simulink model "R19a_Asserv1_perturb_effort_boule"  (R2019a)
settings: Solver=ode15s  StartTime=0.0  StopTime=1  RelTol=1e-3  EnableMultiTasking=on
undefined symbols (not defined in the file): deg, kg, m, manette1_Défaut_sldprt, manette2_Défaut_sldprt, mm, N, rad, s, sigbuilder_block, STL, X, Y, Z
libraries: sm_lib x460, fl_lib x45, nesl_utility x23, simulink x3
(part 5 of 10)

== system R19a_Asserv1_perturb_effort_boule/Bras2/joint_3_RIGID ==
  AXE_BRAS_1_RIGID : Subsystem
  ReferenceFrame : sm_lib/Frames and Transforms/Reference Frame
  Transform : sm_lib/Frames and Transforms/Rigid Transform  TranslationMethod=Cartesian  TranslationStandardOffset=0  TranslationLengthUnit=mm  TranslationStandardAxis=+Z  TranslationCartesianOffset=[-182.62772197331239 126.3991346976174 -143.1183707091507]  TranslationROffset=0  TranslationROffsetUnits=m  TranslationZOffset=0  TranslationZOffsetUnits=m  TranslationThetaOffset=0  TranslationThetaOffsetUnits=deg  RotationMethod=ArbitraryAxis  RotationAngleUnits=rad  RotationStandardAxis=+Z  RotationAngle=2.0943951023931953  RotationArbitraryAxis=[0.57735026918962584 0.57735026918962584 0.57735026918962584]  FollAlignAxisA=+X  BaseAlignAxisA=+Y  FollAlignAxisB=+Y  BaseAlignAxisB=+Z  RotationSequenceAxes=FollowerAxes  RotationSequence=XYX  RotationSequenceAngles=[0 0 0]  RotationSequenceAnglesUnits=deg  RotationMatrix=[1 0 0; 0 1 0; 0 0 1]
  Transform1 : sm_lib/Frames and Transforms/Rigid Transform  TranslationMethod=Cartesian  TranslationStandardOffset=0  TranslationLengthUnit=mm  TranslationStandardAxis=+Z  TranslationCartesianOffset=[-181.62772197331239 116.1902983931664 -133.8263224253264]  TranslationROffset=0  TranslationROffsetUnits=m  TranslationZOffset=0  TranslationZOffsetUnits=m  TranslationThetaOffset=0  TranslationThetaOffsetUnits=deg  RotationMethod=ArbitraryAxis  RotationAngleUnits=rad  RotationStandardAxis=+Z  RotationAngle=1.9754511492118267  RotationArbitraryAxis=[-0.53149434051907762 -0.5314943405190774 -0.65956616953296032]  FollAlignAxisA=+X  BaseAlignAxisA=+Y  FollAlignAxisB=+Y  BaseAlignAxisB=+Z  RotationSequenceAxes=FollowerAxes  RotationSequence=XYX  RotationSequenceAngles=[0 0 0]  RotationSequenceAnglesUnits=deg  RotationMatrix=[1 0 0; 0 1 0; 0 0 1]
  Transform2 : sm_lib/Frames and Transforms/Rigid Transform  TranslationMethod=Cartesian  TranslationStandardOffset=0  TranslationLengthUnit=mm  TranslationStandardAxis=+Z  TranslationCartesianOffset=[-153.62772197331239 116.19029839316639 -133.82632242532642]  TranslationROffset=0  TranslationROffsetUnits=m  TranslationZOffset=0  TranslationZOffsetUnits=m  TranslationThetaOffset=0  TranslationThetaOffsetUnits=deg  RotationMethod=ArbitraryAxis  RotationAngleUnits=rad  RotationStandardAxis=+Z  RotationAngle=1.9754511492118267  RotationArbitraryAxis=[-0.53149434051907762 -0.5314943405190774 -0.65956616953296032]  FollAlignAxisA=+X  BaseAlignAxisA=+Y  FollAlignAxisB=+Y  BaseAlignAxisB=+Z  RotationSequenceAxes=FollowerAxes  RotationSequence=XYX  RotationSequenceAngles=[0 0 0]  RotationSequenceAnglesUnits=deg  RotationMatrix=[1 0 0; 0 1 0; 0 0 1]
  Transform3 : sm_lib/Frames and Transforms/Rigid Transform  TranslationMethod=Cartesian  TranslationStandardOffset=0  TranslationLengthUnit=mm  TranslationStandardAxis=+Z  TranslationCartesianOffset=[-167.62772197331242 128.09991096385988 -150.93549038919826]  TranslationROffset=0  TranslationROffsetUnits=m  TranslationZOffset=0  TranslationZOffsetUnits=m  TranslationThetaOffset=0  TranslationThetaOffsetUnits=deg  RotationMethod=ArbitraryAxis  RotationAngleUnits=rad  RotationStandardAxis=+Z  RotationAngle=1.7850283121554718  RotationArbitraryAxis=[1 6.7005179906918671e-16 -7.8797744802439854e-16]  FollAlignAxisA=+X  BaseAlignAxisA=+Y  FollAlignAxisB=+Y  BaseAlignAxisB=+Z  RotationSequenceAxes=FollowerAxes  RotationSequence=XYX  RotationSequenceAngles=[0 0 0]  RotationSequenceAnglesUnits=deg  RotationMatrix=[1 0 0; 0 1 0; 0 0 1]
  Transform4 : sm_lib/Frames and Transforms/Rigid Transform  TranslationMethod=Cartesian  TranslationStandardOffset=0  TranslationLengthUnit=mm  TranslationStandardAxis=+Z  TranslationCartesianOffset=[-167.62772197331239 126.3991346976174 -143.1183707091507]  TranslationROffset=0  TranslationROffsetUnits=m  TranslationZOffset=0  TranslationZOffsetUnits=m  TranslationThetaOffset=0  TranslationThetaOffsetUnits=deg  RotationMethod=ArbitraryAxis  RotationAngleUnits=rad  RotationStandardAxis=+Z  RotationAngle=1.5707963267948968  RotationArbitraryAxis=[8.0498418078381935e-17 -1 8.0498418078381935e-17]  FollAlignAxisA=+X  BaseAlignAxisA=+Y  FollAlignAxisB=+Y  BaseAlignAxisB=+Z  RotationSequenceAxes=FollowerAxes  RotationSequence=XYX  RotationSequenceAngles=[0 0 0]  RotationSequenceAnglesUnits=deg  RotationMatrix=[1 0 0; 0 1 0; 0 0 1]
  joint_1_RIGID : Subsystem
  F2 : PMIOPort  Side=Left
  F : PMIOPort  Port=2  Side=Right
  F1 : PMIOPort  Port=3  Side=Left
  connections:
  Transform/LConn1 -- ReferenceFrame/RConn1 -- Transform1/LConn1 -- Transform2/LConn1 -- Transform3/LConn1 -- Transform4/LConn1
  Transform/RConn1 -- F/RConn1
  Transform1/RConn1 -- F1/RConn1
  Transform2/RConn1 -- F2/RConn1
  Transform3/RConn1 -- joint_1_RIGID/LConn1
  AXE_BRAS_1_RIGID/LConn1 -- Transform4/RConn1

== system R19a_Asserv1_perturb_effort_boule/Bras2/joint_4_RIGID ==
  AXE_BRAS_1_RIGID : Subsystem
  ReferenceFrame : sm_lib/Frames and Transforms/Reference Frame
  Transform : sm_lib/Frames and Transforms/Rigid Transform  TranslationMethod=Cartesian  TranslationStandardOffset=0  TranslationLengthUnit=mm  TranslationStandardAxis=+Z  TranslationCartesianOffset=[-177.62772197331228 126.39913469764599 -143.11837070916687]  TranslationROffset=0  TranslationROffsetUnits=m  TranslationZOffset=0  TranslationZOffsetUnits=m  TranslationThetaOffset=0  TranslationThetaOffsetUnits=deg  RotationMethod=ArbitraryAxis  RotationAngleUnits=rad  RotationStandardAxis=+Z  RotationAngle=2.0943951023931962  RotationArbitraryAxis=[0.5773502691896254 0.57735026918962584 0.57735026918962595]  FollAlignAxisA=+X  BaseAlignAxisA=+Y  FollAlignAxisB=+Y  BaseAlignAxisB=+Z  RotationSequenceAxes=FollowerAxes  RotationSequence=XYX  RotationSequenceAngles=[0 0 0]  RotationSequenceAnglesUnits=deg  RotationMatrix=[1 0 0; 0 1 0; 0 0 1]
  Transform1 : sm_lib/Frames and Transforms/Rigid Transform  TranslationMethod=Cartesian  TranslationStandardOffset=0  TranslationLengthUnit=mm  TranslationStandardAxis=+Z  TranslationCartesianOffset=[-181.6277219733183 116.19029839316549 -133.82632242532227]  TranslationROffset=0  TranslationROffsetUnits=m  TranslationZOffset=0  TranslationZOffsetUnits=m  TranslationThetaOffset=0  TranslationThetaOffsetUnits=deg  RotationMethod=ArbitraryAxis  RotationAngleUnits=rad  RotationStandardAxis=+Z  RotationAngle=1.9754511492118263  RotationArbitraryAxis=[-0.53149434051907762 -0.53149434051907762 -0.6595661695329601]  FollAlignAxisA=+X  BaseAlignAxisA=+Y  FollAlignAxisB=+Y  BaseAlignAxisB=+Z  RotationSequenceAxes=FollowerAxes  RotationSequence=XYX  RotationSequenceAngles=[0 0 0]  RotationSequenceAnglesUnits=deg  RotationMatrix=[1 0 0; 0 1 0; 0 0 1]
  Transform2 : sm_lib/Frames and Transforms/Rigid Transform  TranslationMethod=Cartesian  TranslationStandardOffset=0  TranslationLengthUnit=mm  TranslationStandardAxis=+Z  TranslationCartesianOffset=[-153.62772197331839 131.82453775326127 -130.42476989284023]  TranslationROffset=0  TranslationROffsetUnits=m  TranslationZOffset=0  TranslationZOffsetUnits=m  TranslationThetaOffset=0  TranslationThetaOffsetUnits=deg  RotationMethod=ArbitraryAxis  RotationAngleUnits=rad  RotationStandardAxis=+Z  RotationAngle=2.2221940470110662  RotationArbitraryAxis=[0.61437017396792992 -0.61437017396793137 0.49507431631748922]  FollAlignAxisA=+X  BaseAlignAxisA=+Y  FollAlignAxisB=+Y  BaseAlignAxisB=+Z  RotationSequenceAxes=FollowerAxes  RotationSequence=XYX  RotationSequenceAngles=[0 0 0]  RotationSequenceAnglesUnits=deg  RotationMatrix=[1 0 0; 0 1 0; 0 0 1]
  Transform3 : sm_lib/Frames and Transforms/Rigid Transform  TranslationMethod=Cartesian  TranslationStandardOffset=0  TranslationLengthUnit=mm  TranslationStandardAxis=+Z  TranslationCartesianOffset=[-167.62772197331242 128.09991096385986 -150.93549038919815]  TranslationROffset=0  TranslationROffsetUnits=m  TranslationZOffset=0  TranslationZOffsetUnits=m  TranslationThetaOffset=0  TranslationThetaOffsetUnits=deg  RotationMethod=ArbitraryAxis  RotationAngleUnits=rad  RotationStandardAxis=+Z  RotationAngle=1.785028312155472  RotationArbitraryAxis=[1 8.8696087027513098e-16 -7.493533857789905e-16]  FollAlignAxisA=+X  BaseAlignAxisA=+Y  FollAlignAxisB=+Y  BaseAlignAxisB=+Z  RotationSequenceAxes=FollowerAxes  RotationSequence=XYX  RotationSequenceAngles=[0 0 0]  RotationSequenceAnglesUnits=deg  RotationMatrix=[1 0 0; 0 1 0; 0 0 1]
  Transform4 : sm_lib/Frames and Transforms/Rigid Transform  TranslationMethod=Cartesian  TranslationStandardOffset=0  TranslationLengthUnit=mm  TranslationStandardAxis=+Z  TranslationCartesianOffset=[-167.62772197331239 126.39913469761737 -143.11837070915061]  TranslationROffset=0  TranslationROffsetUnits=m  TranslationZOffset=0  TranslationZOffsetUnits=m  TranslationThetaOffset=0  TranslationThetaOffsetUnits=deg  RotationMethod=ArbitraryAxis  RotationAngleUnits=rad  RotationStandardAxis=+Z  RotationAngle=1.570796326794897  RotationArbitraryAxis=[-0 -1 -0]  FollAlignAxisA=+X  BaseAlignAxisA=+Y  FollAlignAxisB=+Y  BaseAlignAxisB=+Z  RotationSequenceAxes=FollowerAxes  RotationSequence=XYX  RotationSequenceAngles=[0 0 0]  RotationSequenceAnglesUnits=deg  RotationMatrix=[1 0 0; 0 1 0; 0 0 1]
  joint_1_RIGID : Subsystem
  F2 : PMIOPort  Side=Right
  F1 : PMIOPort  Port=2  Side=Right
  F : PMIOPort  Port=3  Side=Left
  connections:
  Transform/LConn1 -- ReferenceFrame/RConn1 -- Transform1/LConn1 -- Transform2/LConn1 -- Transform3/LConn1 -- Transform4/LConn1
  Transform/RConn1 -- F/RConn1
  Transform1/RConn1 -- F1/RConn1
  Transform2/RConn1 -- F2/RConn1
  Transform3/RConn1 -- joint_1_RIGID/LConn1
  AXE_BRAS_1_RIGID/LConn1 -- Transform4/RConn1

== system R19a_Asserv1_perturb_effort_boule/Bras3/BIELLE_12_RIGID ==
  AXE_BIELLE_1_RIGID : Subsystem
  AXE_BIELLE_2_RIGID : Subsystem
  BIELLE_PARALLELOGRAMME_1_RIGID : Subsystem
  ReferenceFrame : sm_lib/Frames and Transforms/Reference Frame
  Transform : sm_lib/Frames and Transforms/Rigid Transform  TranslationMethod=Cartesian  TranslationStandardOffset=0  TranslationLengthUnit=mm  TranslationStandardAxis=+Z  TranslationCartesianOffset=[-181.12877100136717 12.999999999999996 -3.249999999999996]  TranslationROffset=0  TranslationROffsetUnits=m  TranslationZOffset=0  TranslationZOffsetUnits=m  TranslationThetaOffset=0  TranslationThetaOffsetUnits=deg  RotationMethod=ArbitraryAxis  RotationAngleUnits=rad  RotationStandardAxis=+Z  RotationAngle=2.0943951023931953  RotationArbitraryAxis=[0.57735026918962584 -0.57735026918962584 0.57735026918962584]  FollAlignAxisA=+X  BaseAlignAxisA=+Y  FollAlignAxisB=+Y  BaseAlignAxisB=+Z  RotationSequenceAxes=FollowerAxes  RotationSequence=XYX  RotationSequenceAngles=[0 0 0]  RotationSequenceAnglesUnits=deg  RotationMatrix=[1 0 0; 0 1 0; 0 0 1]
  Transform1 : sm_lib/Frames and Transforms/Rigid Transform  TranslationMethod=Cartesian  TranslationStandardOffset=0  TranslationLengthUnit=mm  TranslationStandardAxis=+Z  TranslationCartesianOffset=[-181.1287710013672 12.999999999999963 -105.75000000000004]  TranslationROffset=0  TranslationROffsetUnits=m  TranslationZOffset=0  TranslationZOffsetUnits=m  TranslationThetaOffset=0  TranslationThetaOffsetUnits=deg  RotationMethod=ArbitraryAxis  RotationAngleUnits=rad  RotationStandardAxis=+Z  RotationAngle=2.0943951023931957  RotationArbitraryAxis=[0.57735026918962573 -0.57735026918962573 0.57735026918962562]  FollAlignAxisA=+X  BaseAlignAxisA=+Y  FollAlignAxisB=+Y  BaseAlignAxisB=+Z  RotationSequenceAxes=FollowerAxes  RotationSequence=XYX  RotationSequenceAngles=[0 0 0]  RotationSequenceAnglesUnits=deg  RotationMatrix=[1 0 0; 0 1 0; 0 0 1]
  Transform2 : sm_lib/Frames and Transforms/Rigid Transform  TranslationMethod=Cartesian  TranslationStandardOffset=0  TranslationLengthUnit=mm  TranslationStandardAxis=+Z  TranslationCartesianOffset=[-178.12877100136717 4.9999999999999902 -54.500000000000021]  TranslationROffset=0  TranslationROffsetUnits=m  TranslationZOffset=0  TranslationZOffsetUnits=m  TranslationThetaOffset=0  TranslationThetaOffsetUnits=deg  RotationMethod=ArbitraryAxis  RotationAngleUnits=rad  RotationStandardAxis=+Z  RotationAngle=3.1415926535897931  RotationArbitraryAxis=[-0.70710678118654746 0.70710678118654757 0]  FollAlignAxisA=+X  BaseAlignAxisA=+Y  FollAlignAxisB=+Y  BaseAlignAxisB=+Z  RotationSequenceAxes=FollowerAxes  RotationSequence=XYX  RotationSequenceAngles=[0 0 0]  RotationSequenceAnglesUnits=deg  RotationMatrix=[1 0 0; 0 1 0; 0 0 1]
  Transform3 : sm_lib/Frames and Transforms/Rigid Transform  TranslationMethod=Cartesian  TranslationStandardOffset=0  TranslationLengthUnit=mm  TranslationStandardAxis=+Z  TranslationCartesianOffset=[-181.1287710013672 4.9999999999999627 -105.75000000000004]  TranslationROffset=0  TranslationROffsetUnits=m  TranslationZOffset=0  TranslationZOffsetUnits=m  TranslationThetaOffset=0  TranslationThetaOffsetUnits=deg  RotationMethod=ArbitraryAxis  RotationAngleUnits=rad  RotationStandardAxis=+Z  RotationAngle=1.7602050674842991  RotationArbitraryAxis=[-0.82650316451596495 -0.39805308631204944 -0.39805308631204944]  FollAlignAxisA=+X  BaseAlignAxisA=+Y  FollAlignAxisB=+Y  BaseAlignAxisB=+Z  RotationSequenceAxes=FollowerAxes  RotationSequence=XYX  RotationSequenceAngles=[0 0 0]  RotationSequenceAnglesUnits=deg  RotationMatrix=[1 0 0; 0 1 0; 0 0 1]
  Transform4 : sm_lib/Frames and Transforms/Rigid Transform  TranslationMethod=Cartesian  TranslationStandardOffset=0  TranslationLengthUnit=mm  TranslationStandardAxis=+Z  TranslationCartesianOffset=[-181.12877100136717 4.9999999999999902 -3.249999999999996]  TranslationROffset=0  TranslationROffsetUnits=m  TranslationZOffset=0  TranslationZOffsetUnits=m  TranslationThetaOffset=0  TranslationThetaOffsetUnits=deg  RotationMethod=ArbitraryAxis  RotationAngleUnits=rad  RotationStandardAxis=+Z  RotationAngle=1.7602050674842997  RotationArbitraryAxis=[-0.82650316451596506 -0.39805308631204933 -0.39805308631204939]  FollAlignAxisA=+X  BaseAlignAxisA=+Y  FollAlignAxisB=+Y  BaseAlignAxisB=+Z  RotationSequenceAxes=FollowerAxes  RotationSequence=XYX  RotationSequenceAngles=[0 0 0]  RotationSequenceAnglesUnits=deg  RotationMatrix=[1 0 0; 0 1 0; 0 0 1]
  F1 : PMIOPort  Side=Left
  F : PMIOPort  Port=2  Side=Right
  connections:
  Transform/LConn1 -- ReferenceFrame/RConn1 -- Transform1/LConn1 -- Transform2/LConn1 -- Transform3/LConn1 -- Transform4/LConn1
  Transform/RConn1 -- F/RConn1
  Transform1/RConn1 -- F1/RConn1
  BIELLE_PARALLELOGRAMME_1_RIGID/LConn1 -- Transform2/RConn1
  AXE_BIELLE_1_RIGID/LConn1 -- Transform3/RConn1
  AXE_BIELLE_2_RIGID/LConn1 -- Transform4/RConn1

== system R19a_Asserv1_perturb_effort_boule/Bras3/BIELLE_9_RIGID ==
  AXE_BIELLE_1_RIGID : Subsystem
  AXE_BIELLE_2_RIGID : Subsystem
  BIELLE_PARALLELOGRAMME_1_RIGID : Subsystem
  ReferenceFrame : sm_lib/Frames and Transforms/Reference Frame
  Transform : sm_lib/Frames and Transforms/Rigid Transform  TranslationMethod=Cartesian  TranslationStandardOffset=0  TranslationLengthUnit=mm  TranslationStandardAxis=+Z  TranslationCartesianOffset=[-181.12877100136723 12.999999999999982 -105.75000000000001]  TranslationROffset=0  TranslationROffsetUnits=m  TranslationZOffset=0  TranslationZOffsetUnits=m  TranslationThetaOffset=0  TranslationThetaOffsetUnits=deg  RotationMethod=ArbitraryAxis  RotationAngleUnits=rad  RotationStandardAxis=+Z  RotationAngle=2.0943951023931957  RotationArbitraryAxis=[0.57735026918962573 -0.57735026918962573 0.57735026918962562]  FollAlignAxisA=+X  BaseAlignAxisA=+Y  FollAlignAxisB=+Y  BaseAlignAxisB=+Z  RotationSequenceAxes=FollowerAxes  RotationSequence=XYX  RotationSequenceAngles=[0 0 0]  RotationSequenceAnglesUnits=deg  RotationMatrix=[1 0 0; 0 1 0; 0 0 1]
  Transform1 : sm_lib/Frames and Transforms/Rigid Transform  TranslationMethod=Cartesian  TranslationStandardOffset=0  TranslationLengthUnit=mm  TranslationStandardAxis=+Z  TranslationCartesianOffset=[-181.12877100136717 13.000000000000004 -3.2500000000000151]  TranslationROffset=0  TranslationROffsetUnits=m  TranslationZOffset=0  TranslationZOffsetUnits=m  TranslationThetaOffset=0  TranslationThetaOffsetUnits=deg  RotationMethod=ArbitraryAxis  RotationAngleUnits=rad  RotationStandardAxis=+Z  RotationAngle=2.0943951023931957  RotationArbitraryAxis=[0.57735026918962584 -0.57735026918962573 0.57735026918962573]  FollAlignAxisA=+X  BaseAlignAxisA=+Y  FollAlignAxisB=+Y  BaseAlignAxisB=+Z  RotationSequenceAxes=FollowerAxes  RotationSequence=XYX  RotationSequenceAngles=[0 0 0]  RotationSequenceAnglesUnits=deg  RotationMatrix=[1 0 0; 0 1 0; 0 0 1]
  Transform2 : sm_lib/Frames and Transforms/Rigid Transform  TranslationMethod=Cartesian  TranslationStandardOffset=0  TranslationLengthUnit=mm  TranslationStandardAxis=+Z  TranslationCartesianOffset=[-178.12877100136717 5.0000000000000044 -54.500000000000021]  TranslationROffset=0  TranslationROffsetUnits=m  TranslationZOffset=0  TranslationZOffsetUnits=m  TranslationThetaOffset=0  TranslationThetaOffsetUnits=deg  RotationMethod=ArbitraryAxis  RotationAngleUnits=rad  RotationStandardAxis=+Z  RotationAngle=3.1415926535897931  RotationArbitraryAxis=[0.70710678118654746 -0.70710678118654757 3.9252311467094379e-17]  FollAlignAxisA=+X  BaseAlignAxisA=+Y  FollAlignAxisB=+Y  BaseAlignAxisB=+Z  RotationSequenceAxes=FollowerAxes  RotationSequence=XYX  RotationSequenceAngles=[0 0 0]  RotationSequenceAnglesUnits=deg  RotationMatrix=[1 0 0; 0 1 0; 0 0 1]
  Transform3 : sm_lib/Frames and Transforms/Rigid Transform  TranslationMethod=Cartesian  TranslationStandardOffset=0  TranslationLengthUnit=mm  TranslationStandardAxis=+Z  TranslationCartesianOffset=[-181.12877100136723 4.9999999999999902 -105.75000000000001]  TranslationROffset=0  TranslationROffsetUnits=m  TranslationZOffset=0  TranslationZOffsetUnits=m  TranslationThetaOffset=0  TranslationThetaOffsetUnits=deg  RotationMethod=ArbitraryAxis  RotationAngleUnits=rad  RotationStandardAxis=+Z  RotationAngle=1.7602050674842991  RotationArbitraryAxis=[-0.82650316451596495 -0.39805308631204944 -0.39805308631204944]  FollAlignAxisA=+X  BaseAlignAxisA=+Y  FollAlignAxisB=+Y  BaseAlignAxisB=+Z  RotationSequenceAxes=FollowerAxes  RotationSequence=XYX  RotationSequenceAngles=[0 0 0]  RotationSequenceAnglesUnits=deg  RotationMatrix=[1 0 0; 0 1 0; 0 0 1]
  Transform4 : sm_lib/Frames and Transforms/Rigid Transform  TranslationMethod=Cartesian  TranslationStandardOffset=0  TranslationLengthUnit=mm  TranslationStandardAxis=+Z  TranslationCartesianOffset=[-181.12877100136717 5.0000000000000044 -3.2500000000000169]  TranslationROffset=0  TranslationROffsetUnits=m  TranslationZOffset=0  TranslationZOffsetUnits=m  TranslationThetaOffset=0  TranslationThetaOffsetUnits=deg  RotationMethod=ArbitraryAxis  RotationAngleUnits=rad  RotationStandardAxis=+Z  RotationAngle=1.7602050674842993  RotationArbitraryAxis=[-0.82650316451596495 -0.39805308631204939 -0.39805308631204939]  FollAlignAxisA=+X  BaseAlignAxisA=+Y  FollAlignAxisB=+Y  BaseAlignAxisB=+Z  RotationSequenceAxes=FollowerAxes  RotationSequence=XYX  RotationSequenceAngles=[0 0 0]  RotationSequenceAnglesUnits=deg  RotationMatrix=[1 0 0; 0 1 0; 0 0 1]
  F1 : PMIOPort  Side=Left
  F : PMIOPort  Port=2  Side=Right
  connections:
  Transform/LConn1 -- ReferenceFrame/RConn1 -- Transform1/LConn1 -- Transform2/LConn1 -- Transform3/LConn1 -- Transform4/LConn1
  Transform/RConn1 -- F/RConn1
  Transform1/RConn1 -- F1/RConn1
  BIELLE_PARALLELOGRAMME_1_RIGID/LConn1 -- Transform2/RConn1
  AXE_BIELLE_1_RIGID/LConn1 -- Transform3/RConn1
  AXE_BIELLE_2_RIGID/LConn1 -- Transform4/RConn1

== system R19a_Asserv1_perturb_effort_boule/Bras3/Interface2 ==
  Angular Velocity Source : fl_lib/Mechanical/Mechanical Sources/Ideal Angular Velocity Source
  Torque Sensor : fl_lib/Mechanical/Mechanical Sensors/Ideal Torque Sensor
  C : PMIOPort  Side=Left
  T : PMIOPort  Port=2  Side=Right
  w : PMIOPort  Port=3  Side=Right
  R : PMIOPort  Port=4  Side=Left
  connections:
  R/RConn1 -- Angular Velocity Source/LConn1
  Torque Sensor/LConn1 -- Angular Velocity Source/RConn2
  Torque Sensor/RConn2 -- T/RConn1
  C/RConn1 -- Torque Sensor/RConn1
  Angular Velocity Source/RConn1 -- w/RConn1

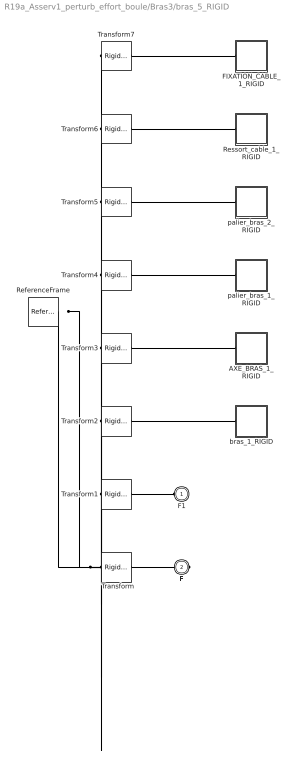
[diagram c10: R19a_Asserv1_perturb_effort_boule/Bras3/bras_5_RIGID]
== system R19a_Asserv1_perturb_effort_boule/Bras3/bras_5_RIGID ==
  AXE_BRAS_1_RIGID : Subsystem
  FIXATION_CABLE_1_RIGID : Subsystem
  ReferenceFrame : sm_lib/Frames and Transforms/Reference Frame
  Ressort_cable_1_RIGID : Subsystem
  Transform : sm_lib/Frames and Transforms/Rigid Transform  TranslationMethod=Cartesian  TranslationStandardOffset=0  TranslationLengthUnit=mm  TranslationStandardAxis=+Z  TranslationCartesianOffset=[-176.59192436800632 99.825618202078189 -20.980989744703674]  TranslationROffset=0  TranslationROffsetUnits=m  TranslationZOffset=0  TranslationZOffsetUnits=m  TranslationThetaOffset=0  TranslationThetaOffsetUnits=deg  RotationMethod=ArbitraryAxis  RotationAngleUnits=rad  RotationStandardAxis=+Z  RotationAngle=2.0943951023931953  RotationArbitraryAxis=[0.57735026918962584 0.57735026918962584 0.57735026918962584]  FollAlignAxisA=+X  BaseAlignAxisA=+Y  FollAlignAxisB=+Y  BaseAlignAxisB=+Z  RotationSequenceAxes=FollowerAxes  RotationSequence=XYX  RotationSequenceAngles=[0 0 0]  RotationSequenceAnglesUnits=deg  RotationMatrix=[1 0 0; 0 1 0; 0 0 1]
  Transform1 : sm_lib/Frames and Transforms/Rigid Transform  TranslationMethod=Cartesian  TranslationStandardOffset=0  TranslationLengthUnit=mm  TranslationStandardAxis=+Z  TranslationCartesianOffset=[-252.36832285678696 39.82561820208025 -20.980989744694625]  TranslationROffset=0  TranslationROffsetUnits=m  TranslationZOffset=0  TranslationZOffsetUnits=m  TranslationThetaOffset=0  TranslationThetaOffsetUnits=deg  RotationMethod=ArbitraryAxis  RotationAngleUnits=rad  RotationStandardAxis=+Z  RotationAngle=2.0943951023931962  RotationArbitraryAxis=[0.57735026918962562 0.57735026918962595 0.57735026918962573]  FollAlignAxisA=+X  BaseAlignAxisA=+Y  FollAlignAxisB=+Y  BaseAlignAxisB=+Z  RotationSequenceAxes=FollowerAxes  RotationSequence=XYX  RotationSequenceAngles=[0 0 0]  RotationSequenceAnglesUnits=deg  RotationMatrix=[1 0 0; 0 1 0; 0 0 1]
  Transform2 : sm_lib/Frames and Transforms/Rigid Transform  TranslationMethod=Cartesian  TranslationStandardOffset=0  TranslationLengthUnit=mm  TranslationStandardAxis=+Z  TranslationCartesianOffset=[-166.59192436800632 39.825618202078182 -20.980989744703674]  TranslationROffset=0  TranslationROffsetUnits=m  TranslationZOffset=0  TranslationZOffsetUnits=m  TranslationThetaOffset=0  TranslationThetaOffsetUnits=deg  RotationMethod=ArbitraryAxis  RotationAngleUnits=rad  RotationStandardAxis=+Z  RotationAngle=1.5707963267948968  RotationArbitraryAxis=[-0 -1 -0]  FollAlignAxisA=+X  BaseAlignAxisA=+Y  FollAlignAxisB=+Y  BaseAlignAxisB=+Z  RotationSequenceAxes=FollowerAxes  RotationSequence=XYX  RotationSequenceAngles=[0 0 0]  RotationSequenceAnglesUnits=deg  RotationMatrix=[1 0 0; 0 1 0; 0 0 1]
  Transform3 : sm_lib/Frames and Transforms/Rigid Transform  TranslationMethod=Cartesian  TranslationStandardOffset=0  TranslationLengthUnit=mm  TranslationStandardAxis=+Z  TranslationCartesianOffset=[-166.59192436800632 39.825618202078182 -20.980989744703674]  TranslationROffset=0  TranslationROffsetUnits=m  TranslationZOffset=0  TranslationZOffsetUnits=m  TranslationThetaOffset=0  TranslationThetaOffsetUnits=deg  RotationMethod=ArbitraryAxis  RotationAngleUnits=rad  RotationStandardAxis=+Z  RotationAngle=1.5707963267948968  RotationArbitraryAxis=[0 1 0]  FollAlignAxisA=+X  BaseAlignAxisA=+Y  FollAlignAxisB=+Y  BaseAlignAxisB=+Z  RotationSequenceAxes=FollowerAxes  RotationSequence=XYX  RotationSequenceAngles=[0 0 0]  RotationSequenceAnglesUnits=deg  RotationMatrix=[1 0 0; 0 1 0; 0 0 1]
  Transform4 : sm_lib/Frames and Transforms/Rigid Transform  TranslationMethod=None  TranslationStandardOffset=0  TranslationLengthUnit=m  TranslationStandardAxis=+Z  TranslationCartesianOffset=[0 0 0]  TranslationROffset=0  TranslationROffsetUnits=m  TranslationZOffset=0  TranslationZOffsetUnits=m  TranslationThetaOffset=0  TranslationThetaOffsetUnits=deg  RotationMethod=None  RotationAngleUnits=deg  RotationStandardAxis=+Z  RotationAngle=0  RotationArbitraryAxis=[0 0 1]  FollAlignAxisA=+X  BaseAlignAxisA=+Y  FollAlignAxisB=+Y  BaseAlignAxisB=+Z  RotationSequenceAxes=FollowerAxes  RotationSequence=XYX  RotationSequenceAngles=[0 0 0]  RotationSequenceAnglesUnits=deg  RotationMatrix=[1 0 0; 0 1 0; 0 0 1]
  Transform5 : sm_lib/Frames and Transforms/Rigid Transform  TranslationMethod=Cartesian  TranslationStandardOffset=0  TranslationLengthUnit=mm  TranslationStandardAxis=+Z  TranslationCartesianOffset=[-333.18384873601264 5.2270863233389884 7.8152493791980202]  TranslationROffset=0  TranslationROffsetUnits=m  TranslationZOffset=0  TranslationZOffsetUnits=m  TranslationThetaOffset=0  TranslationThetaOffsetUnits=deg  RotationMethod=ArbitraryAxis  RotationAngleUnits=rad  RotationStandardAxis=+Z  RotationAngle=3.1415926535897931  RotationArbitraryAxis=[0 0.83121877946981937 -0.55594544755461728]  FollAlignAxisA=+X  BaseAlignAxisA=+Y  FollAlignAxisB=+Y  BaseAlignAxisB=+Z  RotationSequenceAxes=FollowerAxes  RotationSequence=XYX  RotationSequenceAngles=[0 0 0]  RotationSequenceAnglesUnits=deg  RotationMatrix=[1 0 0; 0 1 0; 0 0 1]
  Transform6 : sm_lib/Frames and Transforms/Rigid Transform  TranslationMethod=Cartesian  TranslationStandardOffset=0  TranslationLengthUnit=mm  TranslationStandardAxis=+Z  TranslationCartesianOffset=[-166.59192436800629 17.182941135267082 -24.98098974470367]  TranslationROffset=0  TranslationROffsetUnits=m  TranslationZOffset=0  TranslationZOffsetUnits=m  TranslationThetaOffset=0  TranslationThetaOffsetUnits=deg  RotationMethod=ArbitraryAxis  RotationAngleUnits=rad  RotationStandardAxis=+Z  RotationAngle=1.5707963267948968  RotationArbitraryAxis=[1 0 0]  FollAlignAxisA=+X  BaseAlignAxisA=+Y  FollAlignAxisB=+Y  BaseAlignAxisB=+Z  RotationSequenceAxes=FollowerAxes  RotationSequence=XYX  RotationSequenceAngles=[0 0 0]  RotationSequenceAnglesUnits=deg  RotationMatrix=[1 0 0; 0 1 0; 0 0 1]
  Transform7 : sm_lib/Frames and Transforms/Rigid Transform  TranslationMethod=Cartesian  TranslationStandardOffset=0  TranslationLengthUnit=mm  TranslationStandardAxis=+Z  TranslationCartesianOffset=[-172.59192436800629 90.586314327933948 3.4188407632840221]  TranslationROffset=0  TranslationROffsetUnits=m  TranslationZOffset=0  TranslationZOffsetUnits=m  TranslationThetaOffset=0  TranslationThetaOffsetUnits=deg  RotationMethod=ArbitraryAxis  RotationAngleUnits=rad  RotationStandardAxis=+Z  RotationAngle=1.0159852938148253  RotationArbitraryAxis=[-1 0 0]  FollAlignAxisA=+X  BaseAlignAxisA=+Y  FollAlignAxisB=+Y  BaseAlignAxisB=+Z  RotationSequenceAxes=FollowerAxes  RotationSequence=XYX  RotationSequenceAngles=[0 0 0]  RotationSequenceAnglesUnits=deg  RotationMatrix=[1 0 0; 0 1 0; 0 0 1]
  bras_1_RIGID : Subsystem
  palier_bras_1_RIGID : Subsystem
  palier_bras_2_RIGID : Subsystem
  F1 : PMIOPort  Side=Left
  F : PMIOPort  Port=2  Side=Right
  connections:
  Transform/LConn1 -- ReferenceFrame/RConn1 -- Transform1/LConn1 -- Transform2/LConn1 -- Transform3/LConn1 -- Transform4/LConn1 -- Transform5/LConn1 -- Transform6/LConn1 -- Transform7/LConn1
  Transform/RConn1 -- F/RConn1
  Transform1/RConn1 -- F1/RConn1
  Transform2/RConn1 -- bras_1_RIGID/LConn1
  AXE_BRAS_1_RIGID/LConn1 -- Transform3/RConn1
  Transform4/RConn1 -- palier_bras_1_RIGID/LConn1
  Transform5/RConn1 -- palier_bras_2_RIGID/LConn1
  Ressort_cable_1_RIGID/LConn1 -- Transform6/RConn1
  FIXATION_CABLE_1_RIGID/LConn1 -- Transform7/RConn1

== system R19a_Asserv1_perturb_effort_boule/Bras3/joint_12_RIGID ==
  AXE_BRAS_1_RIGID : Subsystem
  ReferenceFrame : sm_lib/Frames and Transforms/Reference Frame
  Transform : sm_lib/Frames and Transforms/Rigid Transform  TranslationMethod=Cartesian  TranslationStandardOffset=0  TranslationLengthUnit=mm  TranslationStandardAxis=+Z  TranslationCartesianOffset=[-181.62772197331543 131.82453775326098 -130.42476989283941]  TranslationROffset=0  TranslationROffsetUnits=m  TranslationZOffset=0  TranslationZOffsetUnits=m  TranslationThetaOffset=0  TranslationThetaOffsetUnits=deg  RotationMethod=ArbitraryAxis  RotationAngleUnits=rad  RotationStandardAxis=+Z  RotationAngle=2.2221940470110657  RotationArbitraryAxis=[0.61437017396793003 -0.61437017396793026 0.49507431631749033]  FollAlignAxisA=+X  BaseAlignAxisA=+Y  FollAlignAxisB=+Y  BaseAlignAxisB=+Z  RotationSequenceAxes=FollowerAxes  RotationSequence=XYX  RotationSequenceAngles=[0 0 0]  RotationSequenceAnglesUnits=deg  RotationMatrix=[1 0 0; 0 1 0; 0 0 1]
  Transform1 : sm_lib/Frames and Transforms/Rigid Transform  TranslationMethod=Cartesian  TranslationStandardOffset=0  TranslationLengthUnit=mm  TranslationStandardAxis=+Z  TranslationCartesianOffset=[-177.62772197331262 126.39913469758682 -143.11837070913361]  TranslationROffset=0  TranslationROffsetUnits=m  TranslationZOffset=0  TranslationZOffsetUnits=m  TranslationThetaOffset=0  TranslationThetaOffsetUnits=deg  RotationMethod=ArbitraryAxis  RotationAngleUnits=rad  RotationStandardAxis=+Z  RotationAngle=2.0943951023931953  RotationArbitraryAxis=[0.57735026918962595 0.57735026918962584 0.57735026918962562]  FollAlignAxisA=+X  BaseAlignAxisA=+Y  FollAlignAxisB=+Y  BaseAlignAxisB=+Z  RotationSequenceAxes=FollowerAxes  RotationSequence=XYX  RotationSequenceAngles=[0 0 0]  RotationSequenceAnglesUnits=deg  RotationMatrix=[1 0 0; 0 1 0; 0 0 1]
  Transform2 : sm_lib/Frames and Transforms/Rigid Transform  TranslationMethod=Cartesian  TranslationStandardOffset=0  TranslationLengthUnit=mm  TranslationStandardAxis=+Z  TranslationCartesianOffset=[-153.62772197331537 131.82453775326132 -130.4247698928408]  TranslationROffset=0  TranslationROffsetUnits=m  TranslationZOffset=0  TranslationZOffsetUnits=m  TranslationThetaOffset=0  TranslationThetaOffsetUnits=deg  RotationMethod=ArbitraryAxis  RotationAngleUnits=rad  RotationStandardAxis=+Z  RotationAngle=2.2221940470110662  RotationArbitraryAxis=[0.61437017396793026 -0.61437017396793059 0.49507431631748977]  FollAlignAxisA=+X  BaseAlignAxisA=+Y  FollAlignAxisB=+Y  BaseAlignAxisB=+Z  RotationSequenceAxes=FollowerAxes  RotationSequence=XYX  RotationSequenceAngles=[0 0 0]  RotationSequenceAnglesUnits=deg  RotationMatrix=[1 0 0; 0 1 0; 0 0 1]
  Transform3 : sm_lib/Frames and Transforms/Rigid Transform  TranslationMethod=Cartesian  TranslationStandardOffset=0  TranslationLengthUnit=mm  TranslationStandardAxis=+Z  TranslationCartesianOffset=[-167.62772197331242 128.0999109638598 -150.93549038919824]  TranslationROffset=0  TranslationROffsetUnits=m  TranslationZOffset=0  TranslationZOffsetUnits=m  TranslationThetaOffset=0  TranslationThetaOffsetUnits=deg  RotationMethod=ArbitraryAxis  RotationAngleUnits=rad  RotationStandardAxis=+Z  RotationAngle=1.7850283121554718  RotationArbitraryAxis=[1 8.3181277610745589e-16 -6.6018680201685363e-16]  FollAlignAxisA=+X  BaseAlignAxisA=+Y  FollAlignAxisB=+Y  BaseAlignAxisB=+Z  RotationSequenceAxes=FollowerAxes  RotationSequence=XYX  RotationSequenceAngles=[0 0 0]  RotationSequenceAnglesUnits=deg  RotationMatrix=[1 0 0; 0 1 0; 0 0 1]
  Transform4 : sm_lib/Frames and Transforms/Rigid Transform  TranslationMethod=Cartesian  TranslationStandardOffset=0  TranslationLengthUnit=mm  TranslationStandardAxis=+Z  TranslationCartesianOffset=[-167.62772197331242 126.39913469761733 -143.11837070915067]  TranslationROffset=0  TranslationROffsetUnits=m  TranslationZOffset=0  TranslationZOffsetUnits=m  TranslationThetaOffset=0  TranslationThetaOffsetUnits=deg  RotationMethod=ArbitraryAxis  RotationAngleUnits=rad  RotationStandardAxis=+Z  RotationAngle=1.5707963267948968  RotationArbitraryAxis=[5.5511151231257809e-17 -1 -5.5511151231257809e-17]  FollAlignAxisA=+X  BaseAlignAxisA=+Y  FollAlignAxisB=+Y  BaseAlignAxisB=+Z  RotationSequenceAxes=FollowerAxes  RotationSequence=XYX  RotationSequenceAngles=[0 0 0]  RotationSequenceAnglesUnits=deg  RotationMatrix=[1 0 0; 0 1 0; 0 0 1]
  joint_1_RIGID : Subsystem
  F2 : PMIOPort  Side=Right
  F1 : PMIOPort  Port=2  Side=Left
  F : PMIOPort  Port=3  Side=Right
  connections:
  Transform/LConn1 -- ReferenceFrame/RConn1 -- Transform1/LConn1 -- Transform2/LConn1 -- Transform3/LConn1 -- Transform4/LConn1
  Transform/RConn1 -- F/RConn1
  Transform1/RConn1 -- F1/RConn1
  Transform2/RConn1 -- F2/RConn1
  Transform3/RConn1 -- joint_1_RIGID/LConn1
  AXE_BRAS_1_RIGID/LConn1 -- Transform4/RConn1

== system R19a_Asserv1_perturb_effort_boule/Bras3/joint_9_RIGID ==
  AXE_BRAS_1_RIGID : Subsystem
  ReferenceFrame : sm_lib/Frames and Transforms/Reference Frame
  Transform : sm_lib/Frames and Transforms/Rigid Transform  TranslationMethod=Cartesian  TranslationStandardOffset=0  TranslationLengthUnit=mm  TranslationStandardAxis=+Z  TranslationCartesianOffset=[-181.62772197330938 116.19029839316687 -133.82632242532907]  TranslationROffset=0  TranslationROffsetUnits=m  TranslationZOffset=0  TranslationZOffsetUnits=m  TranslationThetaOffset=0  TranslationThetaOffsetUnits=deg  RotationMethod=ArbitraryAxis  RotationAngleUnits=rad  RotationStandardAxis=+Z  RotationAngle=1.9754511492118274  RotationArbitraryAxis=[-0.53149434051907796 -0.53149434051907751 -0.65956616953295999]  FollAlignAxisA=+X  BaseAlignAxisA=+Y  FollAlignAxisB=+Y  BaseAlignAxisB=+Z  RotationSequenceAxes=FollowerAxes  RotationSequence=XYX  RotationSequenceAngles=[0 0 0]  RotationSequenceAnglesUnits=deg  RotationMatrix=[1 0 0; 0 1 0; 0 0 1]
  Transform1 : sm_lib/Frames and Transforms/Rigid Transform  TranslationMethod=Cartesian  TranslationStandardOffset=0  TranslationLengthUnit=mm  TranslationStandardAxis=+Z  TranslationCartesianOffset=[-188.74209771778101 126.39913469761137 -143.11837070916158]  TranslationROffset=0  TranslationROffsetUnits=m  TranslationZOffset=0  TranslationZOffsetUnits=m  TranslationThetaOffset=0  TranslationThetaOffsetUnits=deg  RotationMethod=ArbitraryAxis  RotationAngleUnits=rad  RotationStandardAxis=+Z  RotationAngle=2.0943951023931993  RotationArbitraryAxis=[0.57735026918962373 0.57735026918962706 0.57735026918962651]  FollAlignAxisA=+X  BaseAlignAxisA=+Y  FollAlignAxisB=+Y  BaseAlignAxisB=+Z  RotationSequenceAxes=FollowerAxes  RotationSequence=XYX  RotationSequenceAngles=[0 0 0]  RotationSequenceAnglesUnits=deg  RotationMatrix=[1 0 0; 0 1 0; 0 0 1]
  Transform2 : sm_lib/Frames and Transforms/Rigid Transform  TranslationMethod=Cartesian  TranslationStandardOffset=0  TranslationLengthUnit=mm  TranslationStandardAxis=+Z  TranslationCartesianOffset=[-153.62772197330932 116.19029839316653 -133.82632242532716]  TranslationROffset=0  TranslationROffsetUnits=m  TranslationZOffset=0  TranslationZOffsetUnits=m  TranslationThetaOffset=0  TranslationThetaOffsetUnits=deg  RotationMethod=ArbitraryAxis  RotationAngleUnits=rad  RotationStandardAxis=+Z  RotationAngle=1.9754511492118267  RotationArbitraryAxis=[-0.53149434051907773 -0.53149434051907751 -0.6595661695329601]  FollAlignAxisA=+X  BaseAlignAxisA=+Y  FollAlignAxisB=+Y  BaseAlignAxisB=+Z  RotationSequenceAxes=FollowerAxes  RotationSequence=XYX  RotationSequenceAngles=[0 0 0]  RotationSequenceAnglesUnits=deg  RotationMatrix=[1 0 0; 0 1 0; 0 0 1]
  Transform3 : sm_lib/Frames and Transforms/Rigid Transform  TranslationMethod=Cartesian  TranslationStandardOffset=0  TranslationLengthUnit=mm  TranslationStandardAxis=+Z  TranslationCartesianOffset=[-167.62772197331239 128.09991096385986 -150.93549038919818]  TranslationROffset=0  TranslationROffsetUnits=m  TranslationZOffset=0  TranslationZOffsetUnits=m  TranslationThetaOffset=0  TranslationThetaOffsetUnits=deg  RotationMethod=ArbitraryAxis  RotationAngleUnits=rad  RotationStandardAxis=+Z  RotationAngle=1.785028312155472  RotationArbitraryAxis=[1 8.002259724525313e-16 -6.8382944364994947e-16]  FollAlignAxisA=+X  BaseAlignAxisA=+Y  FollAlignAxisB=+Y  BaseAlignAxisB=+Z  RotationSequenceAxes=FollowerAxes  RotationSequence=XYX  RotationSequenceAngles=[0 0 0]  RotationSequenceAnglesUnits=deg  RotationMatrix=[1 0 0; 0 1 0; 0 0 1]
  Transform4 : sm_lib/Frames and Transforms/Rigid Transform  TranslationMethod=Cartesian  TranslationStandardOffset=0  TranslationLengthUnit=mm  TranslationStandardAxis=+Z  TranslationCartesianOffset=[-167.62772197331236 126.39913469761737 -143.11837070915064]  TranslationROffset=0  TranslationROffsetUnits=m  TranslationZOffset=0  TranslationZOffsetUnits=m  TranslationThetaOffset=0  TranslationThetaOffsetUnits=deg  RotationMethod=ArbitraryAxis  RotationAngleUnits=rad  RotationStandardAxis=+Z  RotationAngle=1.5707963267948968  RotationArbitraryAxis=[-0 -1 -0]  FollAlignAxisA=+X  BaseAlignAxisA=+Y  FollAlignAxisB=+Y  BaseAlignAxisB=+Z  RotationSequenceAxes=FollowerAxes  RotationSequence=XYX  RotationSequenceAngles=[0 0 0]  RotationSequenceAnglesUnits=deg  RotationMatrix=[1 0 0; 0 1 0; 0 0 1]
  joint_1_RIGID : Subsystem
  F2 : PMIOPort  Side=Left
  F : PMIOPort  Port=2  Side=Left
  F1 : PMIOPort  Port=3  Side=Right
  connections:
  Transform/LConn1 -- ReferenceFrame/RConn1 -- Transform1/LConn1 -- Transform2/LConn1 -- Transform3/LConn1 -- Transform4/LConn1
  Transform/RConn1 -- F/RConn1
  Transform1/RConn1 -- F1/RConn1
  Transform2/RConn1 -- F2/RConn1
  Transform3/RConn1 -- joint_1_RIGID/LConn1
  AXE_BRAS_1_RIGID/LConn1 -- Transform4/RConn1

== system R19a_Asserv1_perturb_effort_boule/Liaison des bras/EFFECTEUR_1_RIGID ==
  BASE_1_RIGID : Subsystem
  ReferenceFrame : sm_lib/Frames and Transforms/Reference Frame
  Transform : sm_lib/Frames and Transforms/Rigid Transform  TranslationMethod=Cartesian  TranslationStandardOffset=0  TranslationLengthUnit=mm  TranslationStandardAxis=+Z  TranslationCartesianOffset=[-87.428721422199686 114.78475141038592 178.68957730413138]  TranslationROffset=0  TranslationROffsetUnits=m  TranslationZOffset=0  TranslationZOffsetUnits=m  TranslationThetaOffset=0  TranslationThetaOffsetUnits=deg  RotationMethod=ArbitraryAxis  RotationAngleUnits=rad  RotationStandardAxis=+Z  RotationAngle=1.730474842144561  RotationArbitraryAxis=[0.85183585180135124 0.37038876979862273 0.37038876979861218]  FollAlignAxisA=+X  BaseAlignAxisA=+Y  FollAlignAxisB=+Y  BaseAlignAxisB=+Z  RotationSequenceAxes=FollowerAxes  RotationSequence=XYX  RotationSequenceAngles=[0 0 0]  RotationSequenceAnglesUnits=deg  RotationMatrix=[1 0 0; 0 1 0; 0 0 1]
  Transform1 : sm_lib/Frames and Transforms/Rigid Transform  TranslationMethod=Cartesian  TranslationStandardOffset=0  TranslationLengthUnit=mm  TranslationStandardAxis=+Z  TranslationCartesianOffset=[-45.597843791303056 49.588932155076364 178.68957730412913]  TranslationROffset=0  TranslationROffsetUnits=m  TranslationZOffset=0  TranslationZOffsetUnits=m  TranslationThetaOffset=0  TranslationThetaOffsetUnits=deg  RotationMethod=ArbitraryAxis  RotationAngleUnits=rad  RotationStandardAxis=+Z  RotationAngle=2.2299847707569485  RotationArbitraryAxis=[-0.6163079985177109 -0.49023351775065482 -0.61630799851771478]  FollAlignAxisA=+X  BaseAlignAxisA=+Y  FollAlignAxisB=+Y  BaseAlignAxisB=+Z  RotationSequenceAxes=FollowerAxes  RotationSequence=XYX  RotationSequenceAngles=[0 0 0]  RotationSequenceAnglesUnits=deg  RotationMatrix=[1 0 0; 0 1 0; 0 0 1]
  Transform2 : sm_lib/Frames and Transforms/Rigid Transform  TranslationMethod=Cartesian  TranslationStandardOffset=0  TranslationLengthUnit=mm  TranslationStandardAxis=+Z  TranslationCartesianOffset=[-11.168668790429919 124.06200864616406 178.68957730412961]  TranslationROffset=0  TranslationROffsetUnits=m  TranslationZOffset=0  TranslationZOffsetUnits=m  TranslationThetaOffset=0  TranslationThetaOffsetUnits=deg  RotationMethod=ArbitraryAxis  RotationAngleUnits=rad  RotationStandardAxis=+Z  RotationAngle=2.2733724201793901  RotationArbitraryAxis=[-0.46360505726599749 -0.62652627673442052 0.62652627673442052]  FollAlignAxisA=+X  BaseAlignAxisA=+Y  FollAlignAxisB=+Y  BaseAlignAxisB=+Z  RotationSequenceAxes=FollowerAxes  RotationSequence=XYX  RotationSequenceAngles=[0 0 0]  RotationSequenceAnglesUnits=deg  RotationMatrix=[1 0 0; 0 1 0; 0 0 1]
  Transform3 : sm_lib/Frames and Transforms/Rigid Transform  TranslationMethod=Cartesian  TranslationStandardOffset=0  TranslationLengthUnit=mm  TranslationStandardAxis=+Z  TranslationCartesianOffset=[-18.520156068114318 120.86127823960925 192.68957730412961]  TranslationROffset=0  TranslationROffsetUnits=m  TranslationZOffset=0  TranslationZOffsetUnits=m  TranslationThetaOffset=0  TranslationThetaOffsetUnits=deg  RotationMethod=ArbitraryAxis  RotationAngleUnits=rad  RotationStandardAxis=+Z  RotationAngle=3.141592653589786  RotationArbitraryAxis=[-1 -3.4119484481516466e-30 9.4713860223261135e-16]  FollAlignAxisA=+X  BaseAlignAxisA=+Y  FollAlignAxisB=+Y  BaseAlignAxisB=+Z  RotationSequenceAxes=FollowerAxes  RotationSequence=XYX  RotationSequenceAngles=[0 0 0]  RotationSequenceAnglesUnits=deg  RotationMatrix=[1 0 0; 0 1 0; 0 0 1]
  Transform4 : sm_lib/Frames and Transforms/Rigid Transform  TranslationMethod=Cartesian  TranslationStandardOffset=0  TranslationLengthUnit=mm  TranslationStandardAxis=+Z  TranslationCartesianOffset=[-48.809383170568495 97.91432372411964 187.1895773041295]  TranslationROffset=0  TranslationROffsetUnits=m  TranslationZOffset=0  TranslationZOffsetUnits=m  TranslationThetaOffset=0  TranslationThetaOffsetUnits=deg  RotationMethod=ArbitraryAxis  RotationAngleUnits=rad  RotationStandardAxis=+Z  RotationAngle=0.13705421065001749  RotationArbitraryAxis=[5.1539164000577042e-14 1.7402105179219416e-14 -1]  FollAlignAxisA=+X  BaseAlignAxisA=+Y  FollAlignAxisB=+Y  BaseAlignAxisB=+Z  RotationSequenceAxes=FollowerAxes  RotationSequence=XYX  RotationSequenceAngles=[0 0 0]  RotationSequenceAnglesUnits=deg  RotationMatrix=[1 0 0; 0 1 0; 0 0 1]
  F3 : PMIOPort  Side=Right
  F : PMIOPort  Port=2  Side=Left
  F1 : PMIOPort  Port=3  Side=Left
  F2 : PMIOPort  Port=4  Side=Left
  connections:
  Transform/LConn1 -- ReferenceFrame/RConn1 -- Transform1/LConn1 -- Transform2/LConn1 -- Transform3/LConn1 -- Transform4/LConn1
  Transform/RConn1 -- F/RConn1
  Transform1/RConn1 -- F1/RConn1
  Transform2/RConn1 -- F2/RConn1
  Transform3/RConn1 -- F3/RConn1
  BASE_1_RIGID/LConn1 -- Transform4/RConn1

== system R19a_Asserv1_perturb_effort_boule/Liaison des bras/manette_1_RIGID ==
  ReferenceFrame : sm_lib/Frames and Transforms/Reference Frame
  Transform : sm_lib/Frames and Transforms/Rigid Transform  TranslationMethod=Cartesian  TranslationStandardOffset=0  TranslationLengthUnit=mm  TranslationStandardAxis=+Z  TranslationCartesianOffset=[-33.84478008900291 22.436374240911583 2.2257143640758983]  TranslationROffset=0  TranslationROffsetUnits=m  TranslationZOffset=0  TranslationZOffsetUnits=m  TranslationThetaOffset=0  TranslationThetaOffsetUnits=deg  RotationMethod=ArbitraryAxis  RotationAngleUnits=rad  RotationStandardAxis=+Z  RotationAngle=2.2920311904365782  RotationArbitraryAxis=[0.63063758405056181 -0.45231899713116352 0.63063758405056158]  FollAlignAxisA=+X  BaseAlignAxisA=+Y  FollAlignAxisB=+Y  BaseAlignAxisB=+Z  RotationSequenceAxes=FollowerAxes  RotationSequence=XYX  RotationSequenceAngles=[0 0 0]  RotationSequenceAnglesUnits=deg  RotationMatrix=[1 0 0; 0 1 0; 0 0 1]
  Transform1 : sm_lib/Frames and Transforms/Rigid Transform  TranslationMethod=Cartesian  TranslationStandardOffset=0  TranslationLengthUnit=mm  TranslationStandardAxis=+Z  TranslationCartesianOffset=[-57.010083199545775 -8.8196659542755462 4.7257143640759303]  TranslationROffset=0  TranslationROffsetUnits=m  TranslationZOffset=0  TranslationZOffsetUnits=m  TranslationThetaOffset=0  TranslationThetaOffsetUnits=deg  RotationMethod=ArbitraryAxis  RotationAngleUnits=rad  RotationStandardAxis=+Z  RotationAngle=3.1415926535897931  RotationArbitraryAxis=[-0.15005935073897111 0.98867699035417955 -3.0703282687218866e-18]  FollAlignAxisA=+X  BaseAlignAxisA=+Y  FollAlignAxisB=+Y  BaseAlignAxisB=+Z  RotationSequenceAxes=FollowerAxes  RotationSequence=XYX  RotationSequenceAngles=[0 0 0]  RotationSequenceAnglesUnits=deg  RotationMatrix=[1 0 0; 0 1 0; 0 0 1]
  Transform2 : sm_lib/Frames and Transforms/Rigid Transform  TranslationMethod=Cartesian  TranslationStandardOffset=0  TranslationLengthUnit=mm  TranslationStandardAxis=+Z  TranslationCartesianOffset=[-33.322737031332075 20.894129352085105 2.2257143640758983]  TranslationROffset=0  TranslationROffsetUnits=m  TranslationZOffset=0  TranslationZOffsetUnits=m  TranslationThetaOffset=0  TranslationThetaOffsetUnits=deg  RotationMethod=None  RotationAngleUnits=deg  RotationStandardAxis=+Z  RotationAngle=0  RotationArbitraryAxis=[0 0 1]  FollAlignAxisA=+X  BaseAlignAxisA=+Y  FollAlignAxisB=+Y  BaseAlignAxisB=+Z  RotationSequenceAxes=FollowerAxes  RotationSequence=XYX  RotationSequenceAngles=[0 0 0]  RotationSequenceAnglesUnits=deg  RotationMatrix=[1 0 0; 0 1 0; 0 0 1]
  manette1_1_RIGID : Subsystem
  F : PMIOPort  Side=Right
  F1 : PMIOPort  Port=2  Side=Left
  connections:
  Transform/LConn1 -- ReferenceFrame/RConn1 -- Transform1/LConn1 -- Transform2/LConn1
  Transform/RConn1 -- F/RConn1
  Transform1/RConn1 -- F1/RConn1
  Transform2/RConn1 -- manette1_1_RIGID/LConn1

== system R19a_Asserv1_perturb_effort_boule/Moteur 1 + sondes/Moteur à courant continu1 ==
  note: Kv = 1.18e-1
  Frottement : fl_lib/Mechanical/Rotational Elements/Rotational Friction  brkwy_trq=2.43e-3 N*m  brkwy_vel=0.030296 rad/s  Col_trq=2.43e-3 N*m  visc_coef=2e-6 N*m/(rad/s)  w_specify=off  w_priority=High  w=0 rad/s  w_nominal_specify=off  w_nominal_unit=rad/s  w_nominal_value=1  t_specify=off  t_priority=High  t=0 N*m  t_nominal_specify=off  t_nominal_unit=N*m  t_nominal_value=1
  Inductance induit 35mH : fl_lib/Electrical/Electrical Elements/Inductor  l=35 mH  r=0 Ohm  g=1e-09 1/Ohm  i_specify=off  i_priority=High  i=0 A  i_nominal_specify=off  i_nominal_unit=A  i_nominal_value=1  v_specify=off  v_priority=High  v=0 V  v_nominal_specify=off  v_nominal_unit=V  v_nominal_value=1  i_L_specify=on  i_L_priority=High  i_L=0 A  i_L_nominal_specify=off  i_L_nominal_unit=A  i_L_nominal_value=1
  Inertie Je 10e-6 : fl_lib/Mechanical/Rotational Elements/Inertia  inertia=10.5e-6 kg*m^2  w_specify=on  w_priority=High  w=0 rad/s  w_nominal_specify=off  w_nominal_unit=rad/s  w_nominal_value=1  t_specify=off  t_priority=High  t=0 N*m  t_nominal_specify=off  t_nominal_unit=N*m  t_nominal_value=1
  Moteur parfait : fl_lib/Electrical/Electrical Elements/Rotational Electromechanical Converter  K=1.18e-1 V/(rad/s)  i_specify=off  i_priority=High  i=0 A  i_nominal_specify=off  i_nominal_unit=A  i_nominal_value=1  v_specify=off  v_priority=High  v=0 V  v_nominal_specify=off  v_nominal_unit=V  v_nominal_value=1  t_specify=off  t_priority=High  t=0 N*m  t_nominal_specify=off  t_nominal_unit=N*m  t_nominal_value=1  w_specify=off  w_priority=High  w=0 rad/s  w_nominal_specify=off  w_nominal_unit=rad/s  w_nominal_value=1
  Rinduit 38 Ohms : fl_lib/Electrical/Electrical Elements/Resistor  Tag=Factory Generic  R=38 Ohm  i_specify=off  i_priority=High  i=0 A  i_nominal_specify=off  i_nominal_unit=A  i_nominal_value=1  v_specify=off  v_priority=High  v=0 V  v_nominal_specify=off  v_nominal_unit=V  v_nominal_value=1
  V+ : PMIOPort  Side=Left
  R : PMIOPort  Port=2  Side=Right
  C : PMIOPort  Port=3  Side=Right
  V- : PMIOPort  Port=4  Side=Left
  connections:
  C/RConn1 -- Moteur parfait/RConn2 -- Frottement/RConn1
  R/RConn1 -- Inertie Je 10e-6/LConn1 -- Moteur parfait/LConn2 -- Frottement/LConn1
  Inductance induit 35mH/LConn1 -- Rinduit 38 Ohms/RConn1
  Rinduit 38 Ohms/LConn1 -- V+/RConn1
  V-/RConn1 -- Moteur parfait/RConn1
  Moteur parfait/LConn1 -- Inductance induit 35mH/RConn1

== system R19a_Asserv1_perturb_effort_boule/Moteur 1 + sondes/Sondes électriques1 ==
  " Conv i" : nesl_utility/PS-Simulink Converter  PhysicalDomain=network_engine_domain  SubClassName=ps_output  LeftPortType=input  RightPortType=output  PseudoPeriodic=off  Frequencies=[]  Unit=1  AffineConversion=off
  " Conv v" : nesl_utility/PS-Simulink Converter  PhysicalDomain=network_engine_domain  SubClassName=ps_output  LeftPortType=input  RightPortType=output  PseudoPeriodic=off  Frequencies=[]  Unit=1  AffineConversion=off
  Bras1 : Scope  NumInputPorts=2
  Sonde_I : fl_lib/Electrical/Electrical Sensors/Current Sensor
  Sonde_U : fl_lib/Electrical/Electrical Sensors/Voltage Sensor
  Conn1 : PMIOPort  Side=Left
  Conn2 : PMIOPort  Port=2  Side=Right
  Conn3 : PMIOPort  Port=3  Side=Right
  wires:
  [i] -> Bras1/2  "Imoteur1"
  [u] -> Bras1/1  "Umoteur1"
  " Conv i"/1 -> [i]
  " Conv v"/1 -> [u]
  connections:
  Conn3/RConn1 -- Sonde_U/RConn2
  Conn2/RConn1 -- Sonde_I/RConn2
  Sonde_I/LConn1 -- Sonde_U/LConn1 -- Conn1/RConn1
  Sonde_U/RConn1 -- " Conv v"/LConn1
  Sonde_I/RConn1 -- " Conv i"/LConn1
